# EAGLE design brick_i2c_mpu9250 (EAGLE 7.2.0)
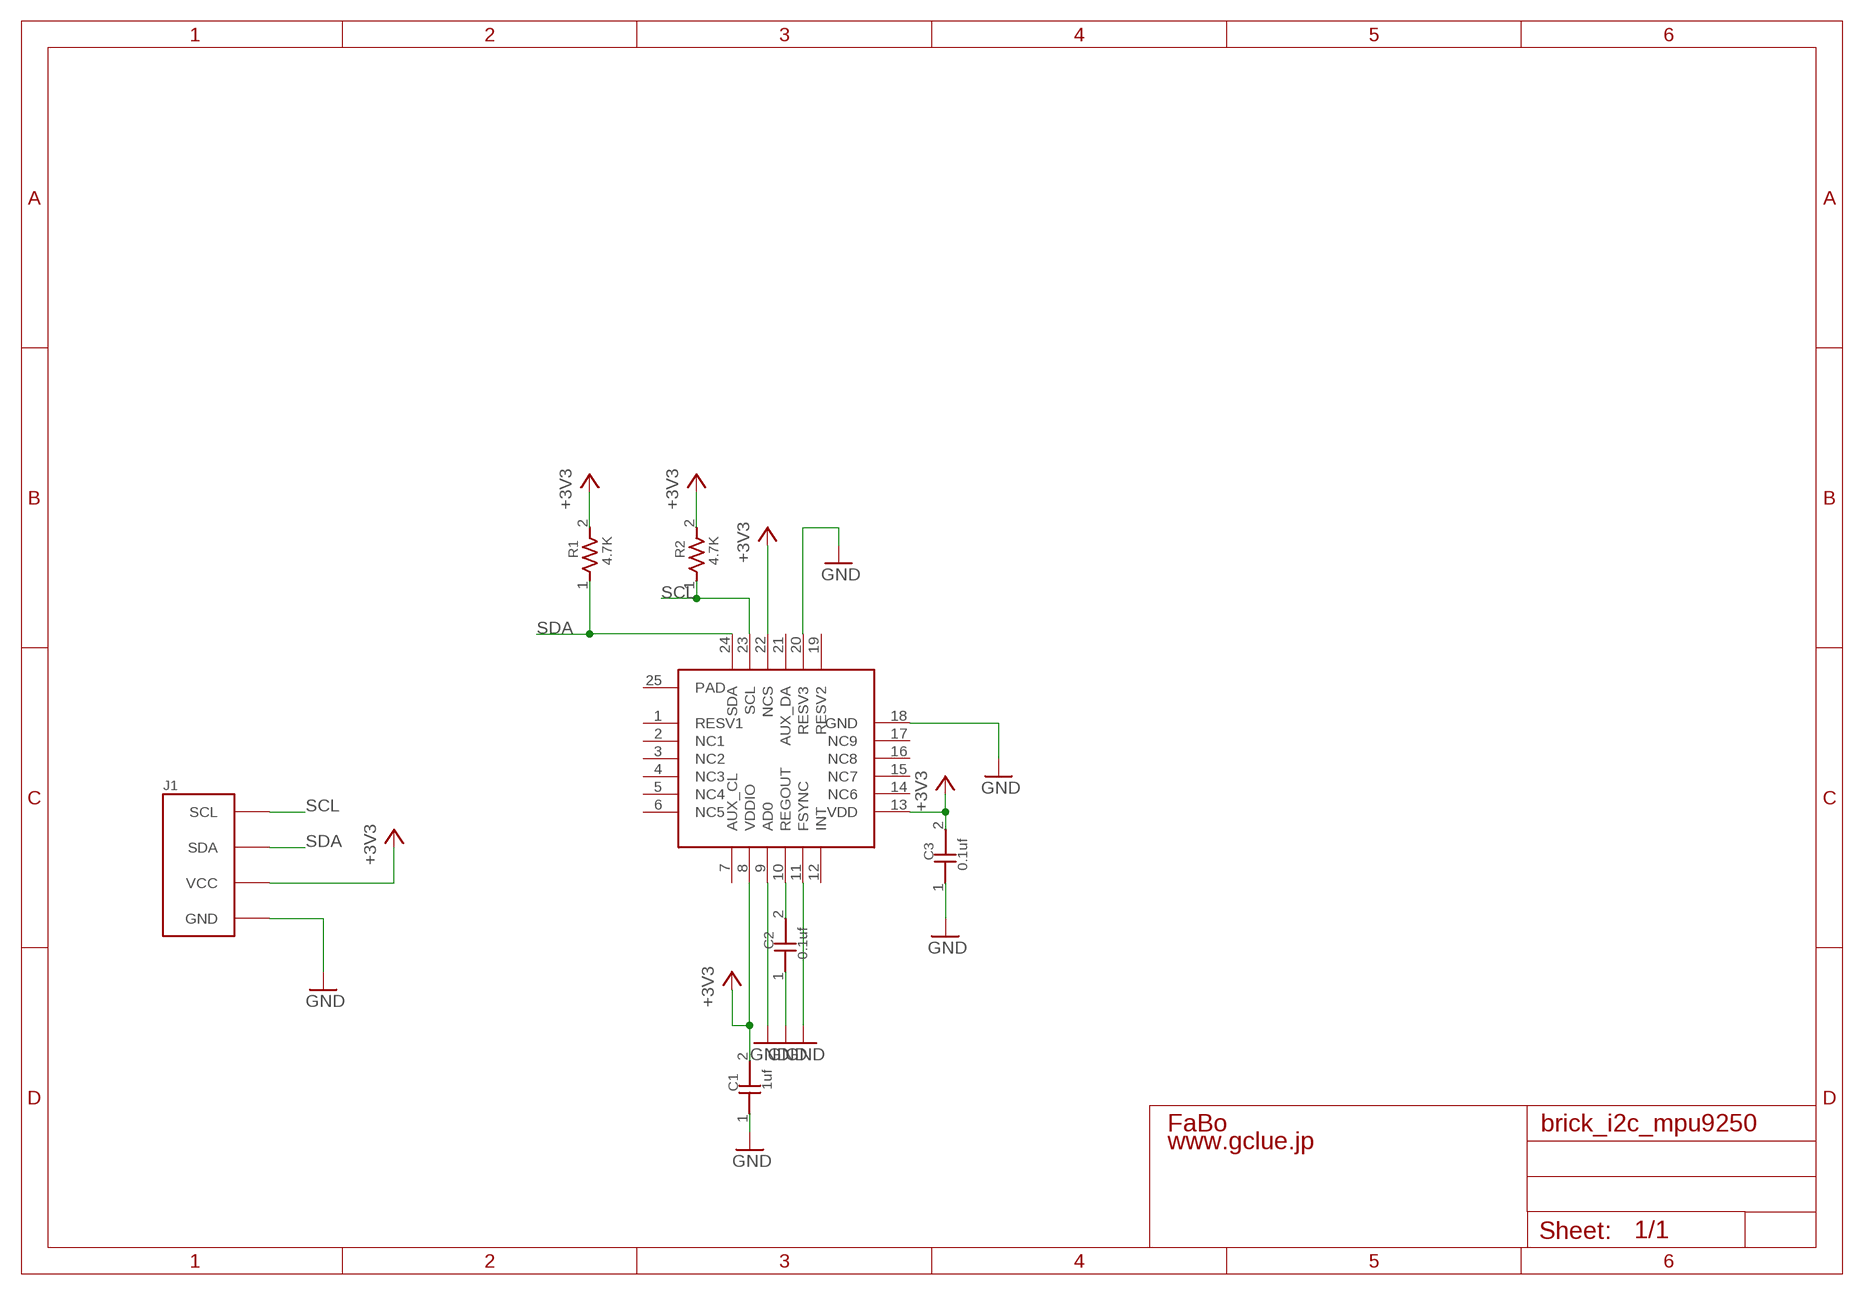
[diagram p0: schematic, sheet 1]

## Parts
C1  1uf  CAPACITOR0603  [0603]
C2  0.1uf  CAPACITOR0603  [0603]
C3  0.1uf  CAPACITOR0603  [0603]
J1  BRICK_I2C  [BRICK_I2C]
R1  4.7K  RESISTOR0603  [0603]
R2  4.7K  RESISTOR0603  [0603]
U$1  INVENSENSE-MPU9250  [LGA-24]

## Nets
+3V3: C1.2 C3.2 J1.VCC R1.2 R2.2 U$1.8(VDDIO) U$1.13(VDD) U$1.22(NCS)
GND: C1.1 C2.1 C3.1 J1.GND U$1.9(AD0) U$1.11(FSYNC) U$1.18(GND) U$1.20(RESV3)
N$3: C2.2 U$1.10(REGOUT)
SCL: J1.SCL R2.1 U$1.23(SCL)
SDA: J1.SDA R1.1 U$1.24(SDA)
Unconnected: U$1.1(RESV1) U$1.2(NC1) U$1.3(NC2) U$1.4(NC3) U$1.5(NC4) U$1.6(NC5) U$1.7(AUX_CL) U$1.12(INT) U$1.14(NC6) U$1.15(NC7) U$1.16(NC8) U$1.17(NC9) U$1.19(RESV2) U$1.21(AUX_DA) U$1.25(PAD)

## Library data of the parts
C1-C3 = GClue-Capacitor:CAPACITOR
J1 = gclue:BRICK_I2C: FaBo Brick 4pin(I2C)
R1 R2 = GClue-Resistors:RESISTOR
U$1 = GClue-Mems:INVENSENSE-MPU9250

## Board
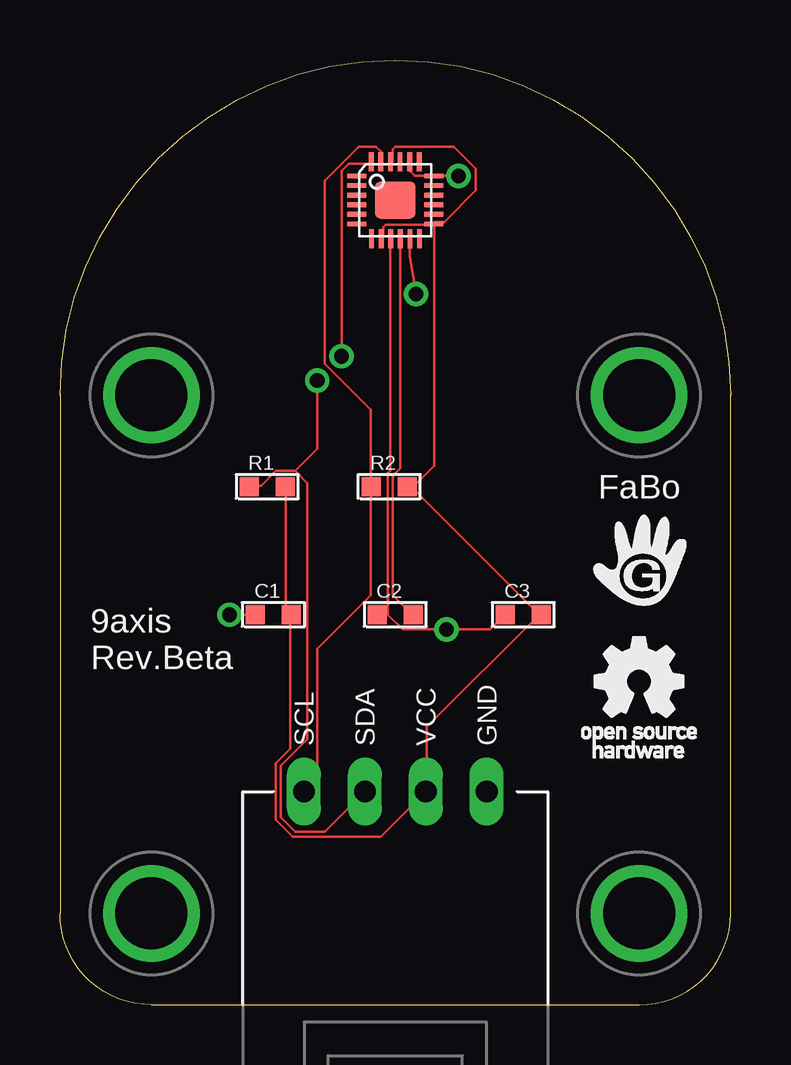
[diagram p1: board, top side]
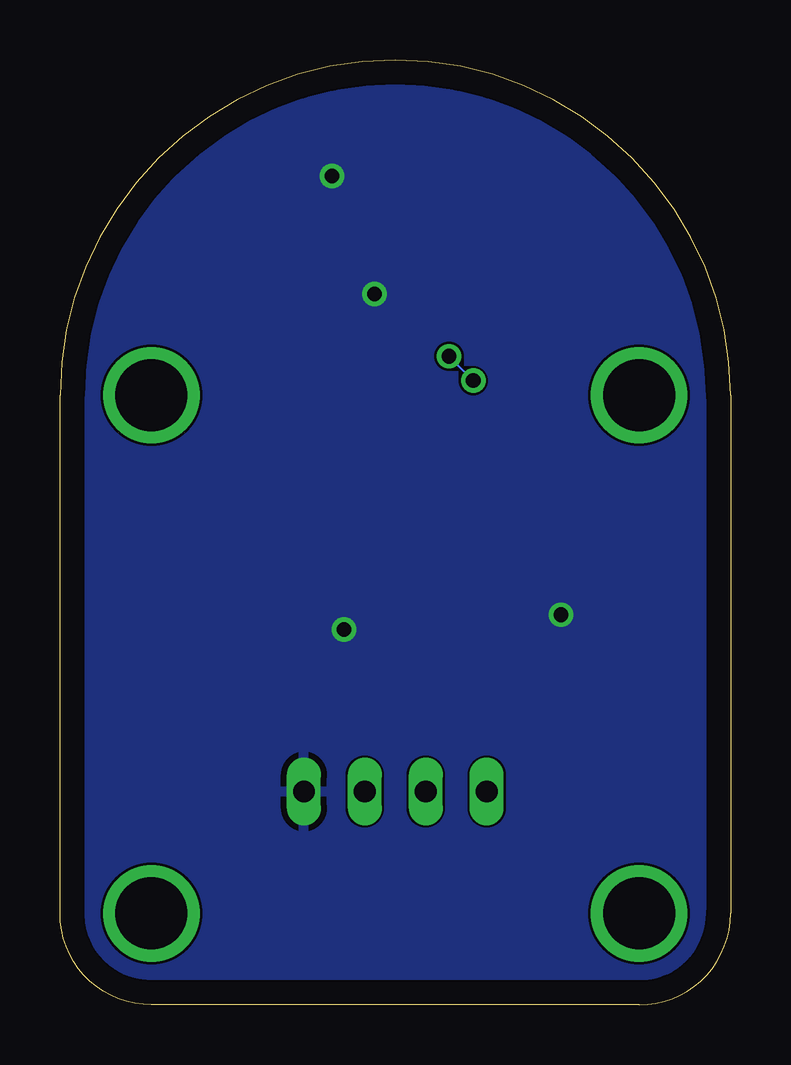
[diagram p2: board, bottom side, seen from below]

Size 27.94 x 39.37 mm. Coordinates in mm from the lower left corner, seen from the top.
Copper layers (1*16): Top 0.035mm / dielectric 1.5mm / Bottom 0.035mm
Design rules "default *": minimum track width 4mil, minimum drill 24mil, track to track 4mil, track to pad 5mil, pad to pad 5mil, via to via 5mil, smd to smd 5mil, copper to edge 40mil, drill to drill 8mil, minimum pad ring 10mil, minimum via ring 8mil, stop-mask expansion 4mil, vias tented up to drill 0mil, thermal gap 10mil

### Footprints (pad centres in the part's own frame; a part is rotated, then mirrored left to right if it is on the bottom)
0603 = smd 0.8 x 0.8: 1 -0.75,0; 2 0.75,0
BRICK_I2C = drill 0.9 long: GND 3.81,-10.16; SCL -3.81,-10.16; SDA -1.27,-10.16; VCC 1.27,-10.16 | drill 3 pad 3.81: P$1 -10.16,6.35; P$2 10.16,6.35; P$3 -10.16,-15.24; P$4 10.16,-15.24
LGA-24 = smd 0.8 x 0.2: 1 -1.6,1.01; 2 -1.6,0.61; 3 -1.6,0.21; 4 -1.6,-0.19; 5 -1.6,-0.59; 6 -1.6,-0.99; 13 1.6,-0.99; 14 1.6,-0.59; 15 1.6,-0.19; 16 1.6,0.21; 17 1.6,0.61; 18 1.6,1.01 | smd 0.2 x 0.8: 7 -0.99,-1.6; 8 -0.59,-1.6; 9 -0.19,-1.6; 10 0.21,-1.6; 11 0.61,-1.6; 12 1.01,-1.6; 19 1,1.6; 20 0.6,1.6; 21 0.2,1.6; 22 -0.2,1.6; 23 -0.6,1.6; 24 -1,1.6 | smd 1.7 x 1.55: 25 0,0

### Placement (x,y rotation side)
C1  8.89,16.26 0 top
C2  13.97,16.26 0 top
C3  19.3,16.26 0 top
J1  13.97,19.05 0 top
R1  8.64,21.59 0 top
R2  13.72,21.59 0 top
U$1  13.97,33.53 0 top
U$3  [LOGO_FABO_M]  24.13,18.54 0 top
U$4  [LOGO_OSHW_T_M]  24.13,13.46 0 top

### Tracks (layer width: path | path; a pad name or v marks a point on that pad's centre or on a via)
+3V3
  Top 0.102: 9.6,16.26 9.4,16.46 9.4,21.54 R1.2 | 9.6,16.26 9.6,10.67 8.99,10.06 8.99,7.72 9.7,7.01 13.36,7.01 J1.VCC 15.29,8.94 15.29,11.58 19.96,16.26 | 9.6,16.26 C1.2 | U$1.8 13.46,32 13.46,32.41 13.56,32.51 15.49,32.51 U$1.13 | U$1.22 13.87,35.15 13.87,35.66 13.97,35.76 16.41,35.76 17.32,34.85 17.32,33.93 16,32.61 15.6,32.61 U$1.13 | 14.68,21.54 14.48,21.54 R2.2 14.68,21.54 | 19.96,16.26 14.68,21.54 | 14.68,21.54 15.6,22.45 15.6,32.51 U$1.13 | 19.96,16.26 C3.2
GND  (via drill 0.61)
  Top 0.102: 13.67,16.26 C2.1 | 13.67,16.26 14.28,15.65 v16.1,15.65 17.93,15.65 C3.1 | 13.67,16.26 13.67,22.15 13.77,22.25 13.77,31.9 U$1.9 | U$1.20 14.58,35.05 14.58,34.75 14.78,34.54 15.49,34.54 U$1.18 15.6,34.54 v16.61,34.54 | v7.06,16.26 C1.1 | v14.83,29.62 14.58,31.19 14.58,31.9 U$1.11
  pour Bottom: 0,0 27.94,0 27.94,39.37 0,39.37
N$3
  Top 0.102: U$1.10 14.17,31.9 14.17,22.35 13.87,22.05 13.87,17.07 14.68,16.26 C2.2
SCL
  Top 0.102: J1.SCL 10.72,9.45 10.72,14.83 12.95,17.07 12.95,21.54 R2.1 12.95,21.64 12.95,24.79 11.02,26.72 11.02,34.34 12.45,35.76 13.16,35.76 13.36,35.56 13.36,35.15 U$1.23
SDA  (via drill 0.61)
  Top 0.102: 9.8,22.25 8.99,22.25 8.38,21.64 7.98,21.64 R1.1 | 9.8,22.25 10.31,21.74 10.31,11.07 9.2,9.96 9.2,7.82 9.8,7.21 11.02,7.21 J1.SDA | v11.74,27.03 11.74,34.75 12.04,35.05 12.95,35.05 U$1.24 | v10.72,26.01 10.72,23.16 9.8,22.25
  Bottom 0.102: v10.72,26.01 v11.74,27.03

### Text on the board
tPlace: 9axis / Rev.Beta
